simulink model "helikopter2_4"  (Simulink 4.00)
settings: Solver=ode1  SolverMode=SingleTasking  StartTime=0.0  StopTime=999999  FixedStep=0.005  MaxStep=10  RelTol=1e-3  AbsTol=1e-3
undefined symbols (not defined in the file or in its folder): simget
libraries: qctools x7

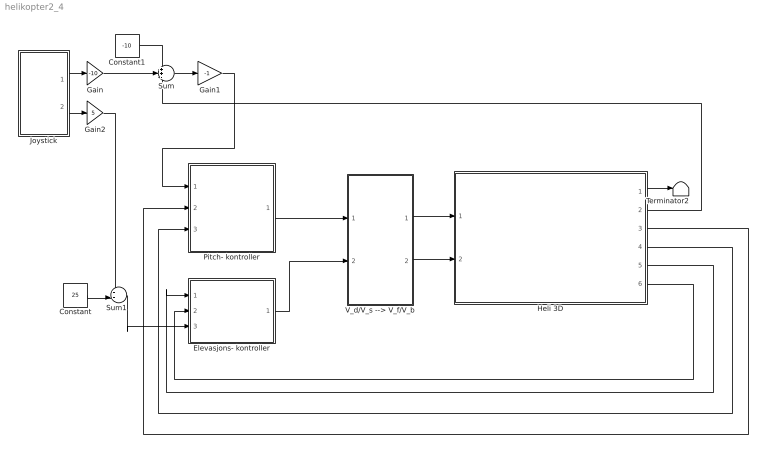
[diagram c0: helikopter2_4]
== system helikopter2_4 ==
  Constant : Constant  Value=25
  Constant1 : Constant  Value=-10
  Elevasjons- kontroller : Subsystem
  Gain : Gain  Gain=-10  Multiplication=Element-wise(K.*u)  SaturateOnIntegerOverflow=on
  Gain1 : Gain  Gain=-1  Multiplication=Element-wise(K.*u)  SaturateOnIntegerOverflow=on
  Gain2 : Gain  Gain=5  Multiplication=Element-wise(K.*u)  SaturateOnIntegerOverflow=on
  Heli 3D : Subsystem
  Joystick : Subsystem
  Pitch- kontroller : Subsystem
  Sum : Sum  Inputs=++-  SaturateOnIntegerOverflow=on
  Sum1 : Sum  Inputs=++|  SaturateOnIntegerOverflow=on
  Terminator2 : Terminator
  V_d/V_s --> V_f/V_b : Subsystem
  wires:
  V_d/V_s --> V_f/V_b/2(V_b) -> Heli 3D/2("V_b, motor bak")
  V_d/V_s --> V_f/V_b/1(V_f) -> Heli 3D/1("V_f, motor foran")
  Pitch- kontroller/1(V_d) -> V_d/V_s --> V_f/V_b/1(V_d)
  Elevasjons- kontroller/1(V_s) -> V_d/V_s --> V_f/V_b/2(V_s)
  Heli 3D/3("Pitch, (grader)") -> Pitch- kontroller/2("p, grader")
  Heli 3D/4("Pitchrate, (grader/sek)") -> Pitch- kontroller/3("p_dot, grader/sek")
  Heli 3D/5("Elevasjon, (grader)") -> Elevasjons- kontroller/1("e, grader")
  Heli 3D/6(Elevasjonsrate (grader/sek)) -> Elevasjons- kontroller/2("e_dot, grader/sek")
  Joystick/1(X Volt) -> Gain/1
  Sum/1 -> Gain1/1
  Gain1/1 -> Pitch- kontroller/1("p_c, grader")
  Heli 3D/1("Vandring, (grader)") -> Terminator2/1
  Sum1/1 -> Elevasjons- kontroller/3("e_c, grader")
  Joystick/2(Y Volt) -> Gain2/1
  Gain2/1 -> Sum1/1
  Heli 3D/2("Vandringsrate, (grader/sek)") -> Sum/3
  Gain/1 -> Sum/2
  Constant1/1 -> Sum/1
  Constant/1 -> Sum1/2

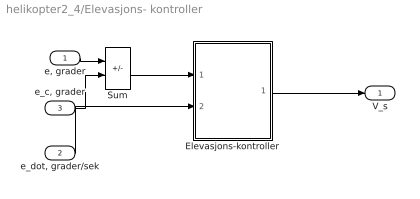
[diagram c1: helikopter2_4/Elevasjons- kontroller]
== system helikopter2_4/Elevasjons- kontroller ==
  "e, grader" : Inport  Port=1  LatchInput=off
  "e_dot, grader/sek" : Inport  Port=2  LatchInput=off
  "e_c, grader" : Inport  Port=3  LatchInput=off
  Elevasjons-kontroller : Subsystem
  Sum : Sum  Inputs=-+  SaturateOnIntegerOverflow=on
  V_s : Outport  Port=1  InitialOutput=0
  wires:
  Sum/1 -> Elevasjons-kontroller/1("e, grader")
  Elevasjons-kontroller/1(out_1) -> V_s/1
  "e, grader"/1 -> Sum/1
  "e_dot, grader/sek"/1 -> Elevasjons-kontroller/2("e, grader/sek")
  "e_c, grader"/1 -> Sum/2

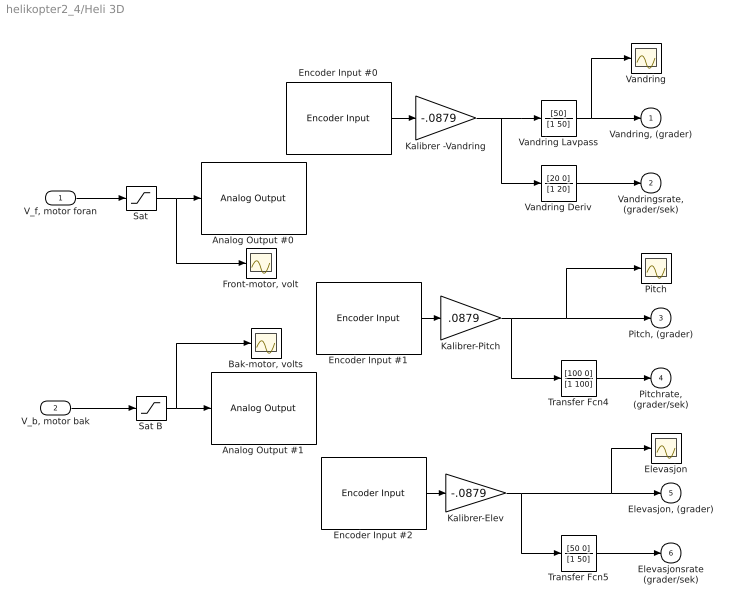
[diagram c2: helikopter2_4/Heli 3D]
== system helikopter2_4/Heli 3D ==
  "V_f, motor foran" : Inport  Port=1  LatchInput=off
  "V_b, motor bak" : Inport  Port=2  LatchInput=off
  Analog Output #0 : qctools/Quanser Consulting MQ3 Series/Analog Output  baseAddr=0x320  channels=0  initialOutputs=0  finalOutputs=0  sampleTime=-1  simulationOutput=off
  Analog Output #1 : qctools/Quanser Consulting MQ3 Series/Analog Output  baseAddr=0x320  channels=1  initialOutputs=0  finalOutputs=0  sampleTime=-1  simulationOutput=off
  "Bak-motor, volts" : Scope
  Elevasjon : Scope
  Encoder Input #0 : qctools/Quanser Consulting MQ3 Series/Encoder Input  baseAddr=0x320  channels=0  initialValues=0  sampleTime=simget(bdroot,'FixedStep')  simulationInput=off
  Encoder Input #1 : qctools/Quanser Consulting MQ3 Series/Encoder Input  baseAddr=0x320  channels=1  initialValues=0  sampleTime=simget(bdroot,'FixedStep')  simulationInput=off
  Encoder Input #2 : qctools/Quanser Consulting MQ3 Series/Encoder Input  baseAddr=0x320  channels=2  initialValues=0  sampleTime=simget(bdroot,'FixedStep')  simulationInput=off
  "Front-motor, volt" : Scope
  Kalibrer -Vandring : Gain  Gain=-.0879  Multiplication=Element-wise(K.*u)  SaturateOnIntegerOverflow=on
  Kalibrer-Elev : Gain  Gain=-.0879  Multiplication=Element-wise(K.*u)  SaturateOnIntegerOverflow=on
  Kalibrer-Pitch : Gain  Gain=.0879  Multiplication=Element-wise(K.*u)  SaturateOnIntegerOverflow=on
  Pitch : Scope
  Sat : Saturate  UpperLimit=5  LowerLimit=-5  LinearizeAsGain=on
  Sat B : Saturate  UpperLimit=5  LowerLimit=-5  LinearizeAsGain=on
  Transfer Fcn4 : TransferFcn  Numerator=[100 0]  Denominator=[1 100]  AbsoluteTolerance=auto  Realization=auto
  Transfer Fcn5 : TransferFcn  Numerator=[50 0]  Denominator=[1 50]  AbsoluteTolerance=auto  Realization=auto
  Vandring : Scope
  Vandring Deriv : TransferFcn  Numerator=[20 0]  Denominator=[1 20]  AbsoluteTolerance=auto  Realization=auto
  Vandring Lavpass : TransferFcn  Numerator=[50]  Denominator=[1 50]  AbsoluteTolerance=auto  Realization=auto
  "Vandring, (grader)" : Outport  Port=1  InitialOutput=0
  "Vandringsrate, (grader/sek)" : Outport  Port=2  InitialOutput=0
  "Pitch, (grader)" : Outport  Port=3  InitialOutput=0
  "Pitchrate, (grader/sek)" : Outport  Port=4  InitialOutput=0
  "Elevasjon, (grader)" : Outport  Port=5  InitialOutput=0
  Elevasjonsrate (grader/sek) : Outport  Port=6  InitialOutput=0
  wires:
  Vandring Deriv/1 -> "Vandringsrate, (grader/sek)"/1
  Vandring Lavpass/1 -> Vandring/1, "Vandring, (grader)"/1
  Encoder Input #0/1 -> Kalibrer -Vandring/1
  Kalibrer -Vandring/1 -> Vandring Deriv/1, Vandring Lavpass/1
  Encoder Input #1/1 -> Kalibrer-Pitch/1
  Kalibrer-Pitch/1 -> Pitch/1, "Pitch, (grader)"/1, Transfer Fcn4/1
  Transfer Fcn4/1 -> "Pitchrate, (grader/sek)"/1
  Encoder Input #2/1 -> Kalibrer-Elev/1
  Kalibrer-Elev/1 -> Transfer Fcn5/1, Elevasjon/1, "Elevasjon, (grader)"/1
  Transfer Fcn5/1 -> Elevasjonsrate (grader/sek)/1
  Sat/1 -> "Front-motor, volt"/1, Analog Output #0/1
  Sat B/1 -> "Bak-motor, volts"/1, Analog Output #1/1
  "V_f, motor foran"/1 -> Sat/1
  "V_b, motor bak"/1 -> Sat B/1

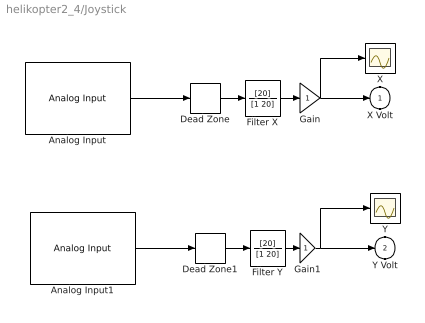
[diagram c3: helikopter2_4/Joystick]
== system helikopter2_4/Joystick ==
  Analog Input : qctools/Quanser Consulting MQ3 Series/Analog Input  baseAddr=0x320  channels=2  sampleTime=simget(bdroot,'FixedStep')  simulationInput=off
  Analog Input1 : qctools/Quanser Consulting MQ3 Series/Analog Input  baseAddr=0x320  channels=3  sampleTime=simget(bdroot,'FixedStep')  simulationInput=off
  Dead Zone : DeadZone  LowerValue=-0.5  UpperValue=0.5  SaturateOnIntegerOverflow=on  LinearizeAsGain=on
  Dead Zone1 : DeadZone  LowerValue=-0.5  UpperValue=0.5  SaturateOnIntegerOverflow=on  LinearizeAsGain=on
  Filter X : TransferFcn  Numerator=[20]  Denominator=[1 20]  AbsoluteTolerance=auto  Realization=auto
  Filter Y : TransferFcn  Numerator=[20]  Denominator=[1 20]  AbsoluteTolerance=auto  Realization=auto
  Gain : Gain  Gain=1  Multiplication=Element-wise(K.*u)  SaturateOnIntegerOverflow=on
  Gain1 : Gain  Gain=1  Multiplication=Element-wise(K.*u)  SaturateOnIntegerOverflow=on
  X : Scope
  Y : Scope
  X Volt : Outport  Port=1  InitialOutput=0
  Y Volt : Outport  Port=2  InitialOutput=0
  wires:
  Dead Zone/1 -> Filter X/1
  Analog Input1/1 -> Dead Zone1/1
  Dead Zone1/1 -> Filter Y/1
  Filter Y/1 -> Gain1/1
  Filter X/1 -> Gain/1
  Analog Input/1 -> Dead Zone/1
  Gain/1 -> X Volt/1, X/1
  Gain1/1 -> Y Volt/1, Y/1

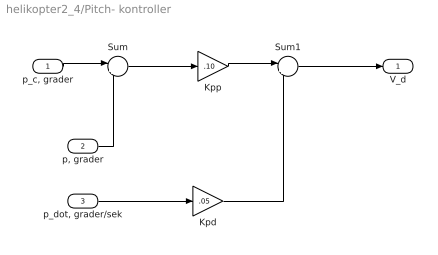
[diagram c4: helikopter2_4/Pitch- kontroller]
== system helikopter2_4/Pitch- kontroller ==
  "p_c, grader" : Inport  Port=1  LatchInput=off
  "p, grader" : Inport  Port=2  LatchInput=off
  "p_dot, grader/sek" : Inport  Port=3  LatchInput=off
  Kpd : Gain  Gain=.05  Multiplication=Element-wise(K.*u)  SaturateOnIntegerOverflow=on
  Kpp : Gain  Gain=.10  Multiplication=Element-wise(K.*u)  SaturateOnIntegerOverflow=on
  Sum : Sum  Inputs=|+-  SaturateOnIntegerOverflow=on
  Sum1 : Sum  Inputs=|+-  SaturateOnIntegerOverflow=on
  V_d : Outport  Port=1  InitialOutput=0
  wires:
  "p_dot, grader/sek"/1 -> Kpd/1
  Sum1/1 -> V_d/1
  Sum/1 -> Kpp/1
  Kpd/1 -> Sum1/2
  "p, grader"/1 -> Sum/2
  "p_c, grader"/1 -> Sum/1
  Kpp/1 -> Sum1/1

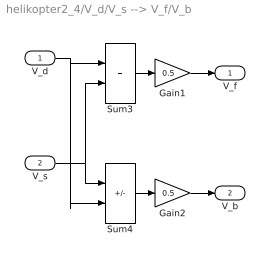
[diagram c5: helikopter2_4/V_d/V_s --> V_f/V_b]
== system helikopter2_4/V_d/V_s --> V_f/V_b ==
  V_d : Inport  Port=1  LatchInput=off
  V_s : Inport  Port=2  LatchInput=off
  Gain1 : Gain  Gain=0.5  Multiplication=Element-wise(K.*u)  SaturateOnIntegerOverflow=on
  Gain2 : Gain  Gain=0.5  Multiplication=Element-wise(K.*u)  SaturateOnIntegerOverflow=on
  Sum3 : Sum  Inputs=++  SaturateOnIntegerOverflow=on
  Sum4 : Sum  Inputs=+-  SaturateOnIntegerOverflow=on
  V_f : Outport  Port=1  InitialOutput=0
  V_b : Outport  Port=2  InitialOutput=0
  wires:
  V_s/1 -> Sum4/1, Sum3/2
  Sum3/1 -> Gain1/1
  Sum4/1 -> Gain2/1
  V_d/1 -> Sum3/1, Sum4/2
  Gain1/1 -> V_f/1
  Gain2/1 -> V_b/1

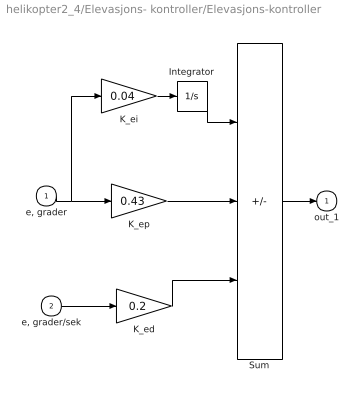
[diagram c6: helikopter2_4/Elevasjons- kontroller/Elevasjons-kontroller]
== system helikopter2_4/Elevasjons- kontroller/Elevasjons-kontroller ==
  "e, grader" : Inport  Port=1  LatchInput=off
  "e, grader/sek" : Inport  Port=2  LatchInput=off
  Integrator : Integrator  ExternalReset=none  InitialConditionSource=internal  InitialCondition=0  LimitOutput=on  UpperSaturationLimit=inf  LowerSaturationLimit=-inf  ShowSaturationPort=off  ShowStatePort=off  AbsoluteTolerance=auto
  K_ed : Gain  Gain=0.2  Multiplication=Element-wise(K.*u)  SaturateOnIntegerOverflow=on
  K_ei : Gain  Gain=0.04  Multiplication=Element-wise(K.*u)  SaturateOnIntegerOverflow=on
  K_ep : Gain  Gain=0.43  Multiplication=Element-wise(K.*u)  SaturateOnIntegerOverflow=on
  Sum : Sum  Inputs=++-  SaturateOnIntegerOverflow=on
  out_1 : Outport  Port=1  InitialOutput=0
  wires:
  K_ei/1 -> Integrator/1
  Integrator/1 -> Sum/1
  Sum/1 -> out_1/1
  "e, grader/sek"/1 -> K_ed/1
  K_ed/1 -> Sum/3
  K_ep/1 -> Sum/2
  "e, grader"/1 -> K_ep/1, K_ei/1
